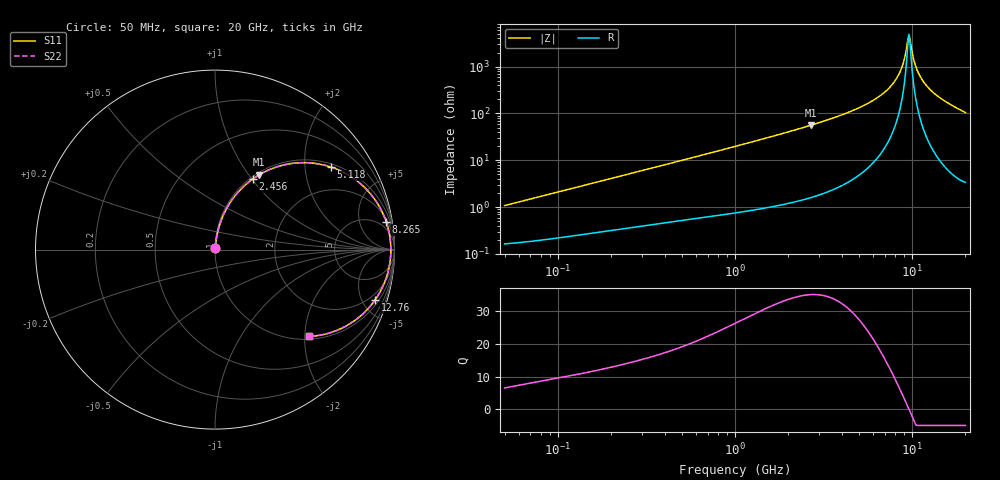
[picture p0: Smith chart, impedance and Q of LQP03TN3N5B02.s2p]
!Murata Part Number: LQP03TN3N5B02
!These Parameters are Measured in Series Mode Connection
!  o--[Z]--o
!Port1  Port2
!  o-------o
!Freq. Start=50[MHz] Stop=20[GHz], 401[Steps]
# Hz S RI R 50
!Freq.(Hz) S11(Real) S11(Imag) S21(Real) S21(Imag) S12(Real) S12(Imag) S22(Real) S22(Imag)
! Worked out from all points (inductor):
!   401 points, 50 MHz to 20 GHz, reference 50 ohm
!   read as one part in series: L = 3.38 nH near 51.52 MHz
!   highest Q = 35.2 at 2.687 GHz (marker M1), where L = 3.33 nH
!   self-resonance near 9.6 GHz
!   S11 on the Smith chart (normalised r, x): 50 MHz: 1.00, +0.02; 2.456 GHz: 1.03, +1.01; 5.118 GHz: 1.10, +2.74; 8.265 GHz: 3, +12; 12.76 GHz: 1.40, -6.24; 20 GHz: 1.07, -2.09
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5e7  0.00175 0.0106  0.9983 -0.0106  0.9983 -0.0106  0.00175 0.0106
1.364002e8  0.00337 0.0281  0.9966 -0.0281  0.9966 -0.0281  0.00337 0.0281
3.721004e8  0.00988 0.0735  0.9901 -0.0735  0.9901 -0.0735  0.00988 0.0735
1e9  0.0442 0.1873  0.9558 -0.1873  0.9558 -0.1873  0.0442 0.1873
2.456456e9  0.2115 0.3943  0.7885 -0.3943  0.7885 -0.3943  0.2115 0.3943
2.687447e9  0.2466 0.417  0.7534 -0.417  0.7534 -0.417  0.2466 0.417
2.728004e9  0.2529 0.4207  0.7471 -0.4207  0.7471 -0.4207  0.2529 0.4207
3.908127e9  0.4494 0.4824  0.5506 -0.4824  0.5506 -0.4824  0.4494 0.4824
5.117541e9  0.6475 0.4595  0.3525 -0.4595  0.3525 -0.4595  0.6475 0.4595
6.311513e9  0.8067 0.3704  0.1933 -0.3704  0.1933 -0.3704  0.8067 0.3704
7.442007e9  0.9096 0.2501  0.0904 -0.2501  0.0904 -0.2501  0.9096 0.2501
8.264682e9  0.9544 0.1538  0.0456 -0.1538  0.0456 -0.1538  0.9544 0.1538
8.774992e9  0.9704 0.0939  0.0296 -0.0939  0.0296 -0.0939  0.9704 0.0939
9.316812e9  0.9787 0.0319  0.0213 -0.0319  0.0213 -0.0319  0.9787 0.0319
9.600142e9  0.9799 0.000425  0.0201 -0.000425  0.0201 -0.000425  0.9799 0.000425
9.745021e9  0.9797 -0.0153  0.0203 0.0153  0.0203 0.0153  0.9797 -0.0153
1.034674e10  0.9738 -0.0782  0.0262 0.0782  0.0262 0.0782  0.9738 -0.0782
1.082228e10  0.9641 -0.1245  0.0359 0.1245  0.0359 0.1245  0.9641 -0.1245
1.166392e10  0.9382 -0.1985  0.0618 0.1985  0.0618 0.1985  0.9382 -0.1985
1.276073e10  0.8926 -0.2795  0.1074 0.2795  0.1074 0.2795  0.8926 -0.2795
1.550395e10  0.7522 -0.4129  0.2478 0.4129  0.2478 0.4129  0.7522 -0.4129
2e10  0.5227 -0.4835  0.4773 0.4835  0.4773 0.4835  0.5227 -0.4835
